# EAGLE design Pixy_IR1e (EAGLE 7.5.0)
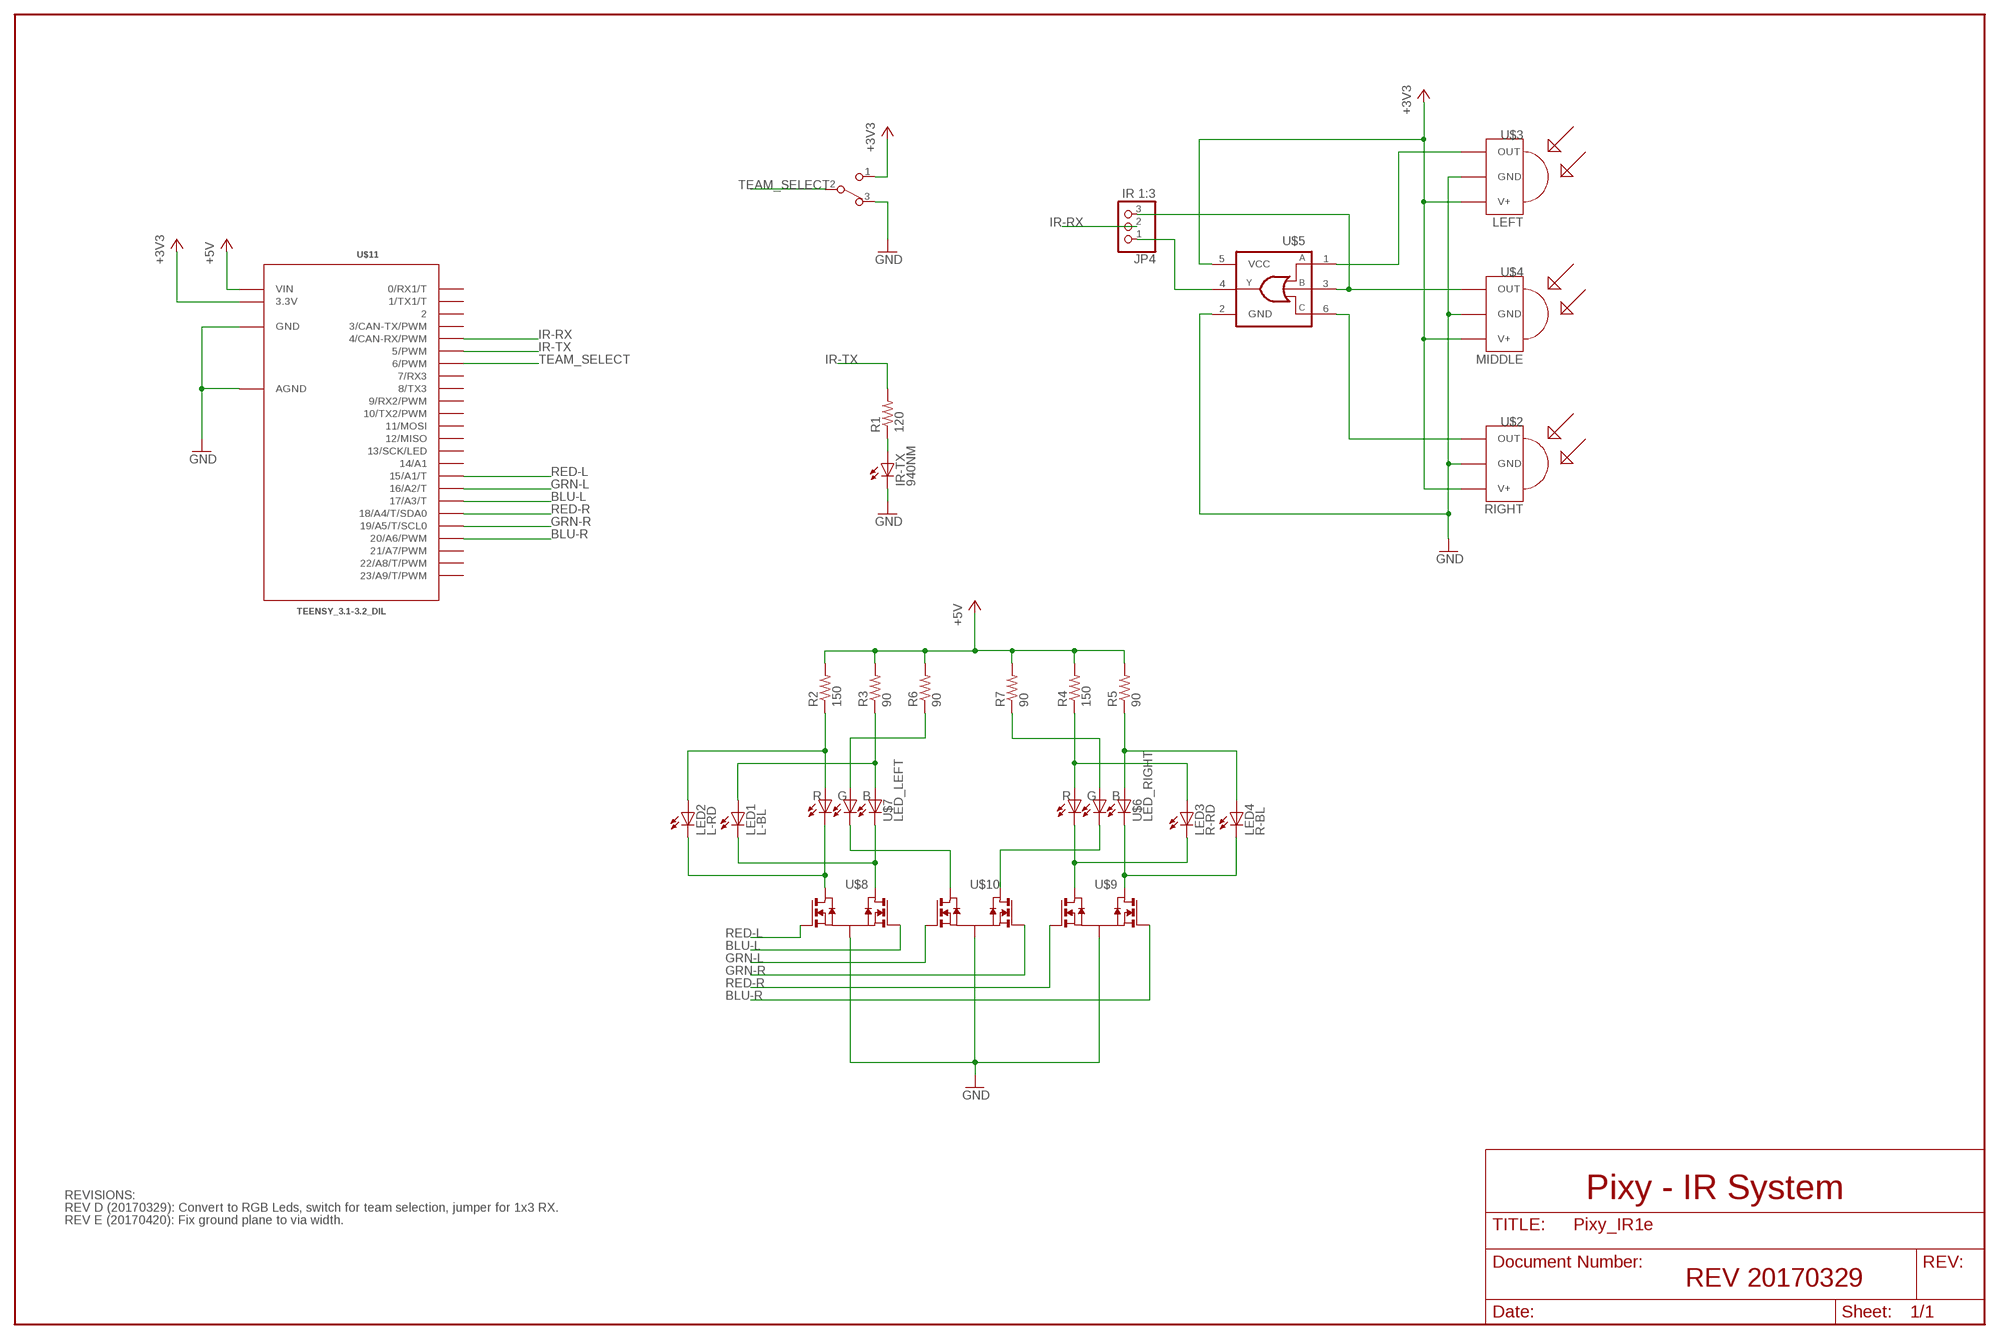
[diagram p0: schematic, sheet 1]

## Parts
IR-TX  940NM  LED5MM  [LED5MM]
JP4  IR 1:3  PINHD-1X3  [1X03]
LED1  L-BL  LED5MM  [LED5MM]
LED2  L-RD  LED5MM  [LED5MM]
LED3  R-RD  LED5MM  [LED5MM]
LED4  R-BL  LED5MM  [LED5MM]
R1  120  R-US_R1206  [R1206]
R2  150  R-US_R1206  [R1206]
R3  90  R-US_R1206  [R1206]
R4  150  R-US_R1206  [R1206]
R5  90  R-US_R1206  [R1206]
R6  90  R-US_R1206  [R1206]
R7  90  R-US_R1206  [R1206]
SW1  TEAM  CAS-120CAS-120B1  [CAS-120B1]
U$2  RIGHT  TSOP3X  [TSOP18XX]
U$3  LEFT  TSOP3X  [TSOP18XX]
U$4  MIDDLE  TSOP3X  [TSOP18XX]
U$5  SN74LVC1G332SOT23-6  [SOT23-6]
U$6  LED_RIGHT  LED_RGB_6SMD  [6-PLCC]
U$7  LED_LEFT  LED_RGB_6SMD  [6-PLCC]
U$8  QS5K2TR  [SOT-23-5]
U$9  QS5K2TR  [SOT-23-5]
U$10  QS5K2TR  [SOT-23-5]
U$11  TEENSY_3.1-3.2_DIL  [TEENSY_3.0-3.2&LC_DIL]

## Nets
+3V3: SW1.1 U$2.VCC(V+) U$3.VCC(V+) U$4.VCC(V+) U$5.5(VCC) U$11.3.3V
+5V: R2.2 R3.2 R4.2 R5.2 R6.2 R7.2 U$11.VIN
BLU-L: U$8.3(G2) U$11.17/A3(17/A3/T)
BLU-R: U$9.3(G2) U$11.20/A6(20/A6/PWM)
GND [ground]: IR-TX.K(C) SW1.3 U$2.GND U$3.GND U$4.GND U$5.2(GND) U$8.2(S) U$9.2(S) U$10.2(S) U$11.AGND U$11.GND
GRN-L: U$10.1(G1) U$11.16/A2(16/A2/T)
GRN-R: U$10.3(G2) U$11.19/A5(19/A5/T/SCL0)
IR-RX: JP4.2 U$11.4(4/CAN-RX/PWM)
IR-TX: R1.2 U$11.5(5/PWM)
N$1: U$2.OUT U$5.6(C)
N$2: U$3.OUT U$5.1(A)
N$3: LED2.A R2.1 U$7.P$1(A1)
N$4: LED1.A R3.1 U$7.P$3(A3)
N$5: R6.1 U$7.P$2(A2)
N$6: U$7.P$5(C2) U$10.5(D1)
N$8: JP4.3 U$4.OUT U$5.3(B)
N$9: JP4.1 U$5.4(Y)
N$10: IR-TX.A R1.1
N$19: LED1.K(C) U$7.P$4(C3) U$8.4(D2)
N$20: LED2.K(C) U$7.P$6(C1) U$8.5(D1)
N$25: LED3.A R4.1 U$6.P$1(A1)
N$26: LED4.A R5.1 U$6.P$3(A3)
N$28: R7.1 U$6.P$2(A2)
N$29: LED3.K(C) U$6.P$6(C1) U$9.5(D1)
N$30: LED4.K(C) U$6.P$4(C3) U$9.4(D2)
N$31: U$6.P$5(C2) U$10.4(D2)
RED-L: U$8.1(G1) U$11.15/A1(15/A1/T)
RED-R: U$9.1(G1) U$11.18/A4(18/A4/T/SDA0)
TEAM_SELECT: SW1.2 U$11.6(6/PWM)
Unconnected: U$11.0(0/RX1/T) U$11.1(1/TX1/T) U$11.2 U$11.3(3/CAN-TX/PWM) U$11.7(7/RX3) U$11.8(8/TX3) U$11.9(9/RX2/PWM) U$11.10(10/TX2/PWM) U$11.11(11/MOSI) U$11.12(12/MISO) U$11.13(13/SCK/LED) U$11.14/A0(14/A1) U$11.21/A7(21/A7/PWM) U$11.22/A8(22/A8/T/PWM) U$11.23/A9(23/A9/T/PWM)

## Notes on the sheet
- REVISIONS: | Pixy - IR System
- REV D (20170329): Convert to RGB Leds, switch for team selection, jumper for 1x3 RX.
- REV E (20170420): Fix ground plane to via width.
- REV 20170329

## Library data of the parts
IR-TX LED1-LED4 = led:LED: LED
JP4 = pinhead:PINHD-1X3: PIN HEADER
R1-R7 = resistor:R-US_: RESISTOR, American symbol
SW1 = Switch2:CAS-120: CAS-120 surface mount type slide switch Producted by COPAL ELECTRONICS Store Information : Digi-Key : http://search.digikey.com/scripts/DkSearch/dksus.dll?Detail&name=CAS120GCT-ND
U$2-U$4 = _Loper:TSOP3X: IR Receiver and Demodulator
U$5 = 74LV:SN74LVC1G332: OR GATE 3-INPUT
U$6 U$7 = _Loper:LED_RGB_6SMD
U$8-U$10 = _Loper:QS5K2TR: MOSFET 2N-CH
U$11 = Teensy_3_and_LC_Series_Boards_v1.4:TEENSY_3.1-3.2_DIL: Teensy 3.1 or 3.2 in a DIL Layout.

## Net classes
0 default: width 0.406 mm
1 ground: width 0.61 mm

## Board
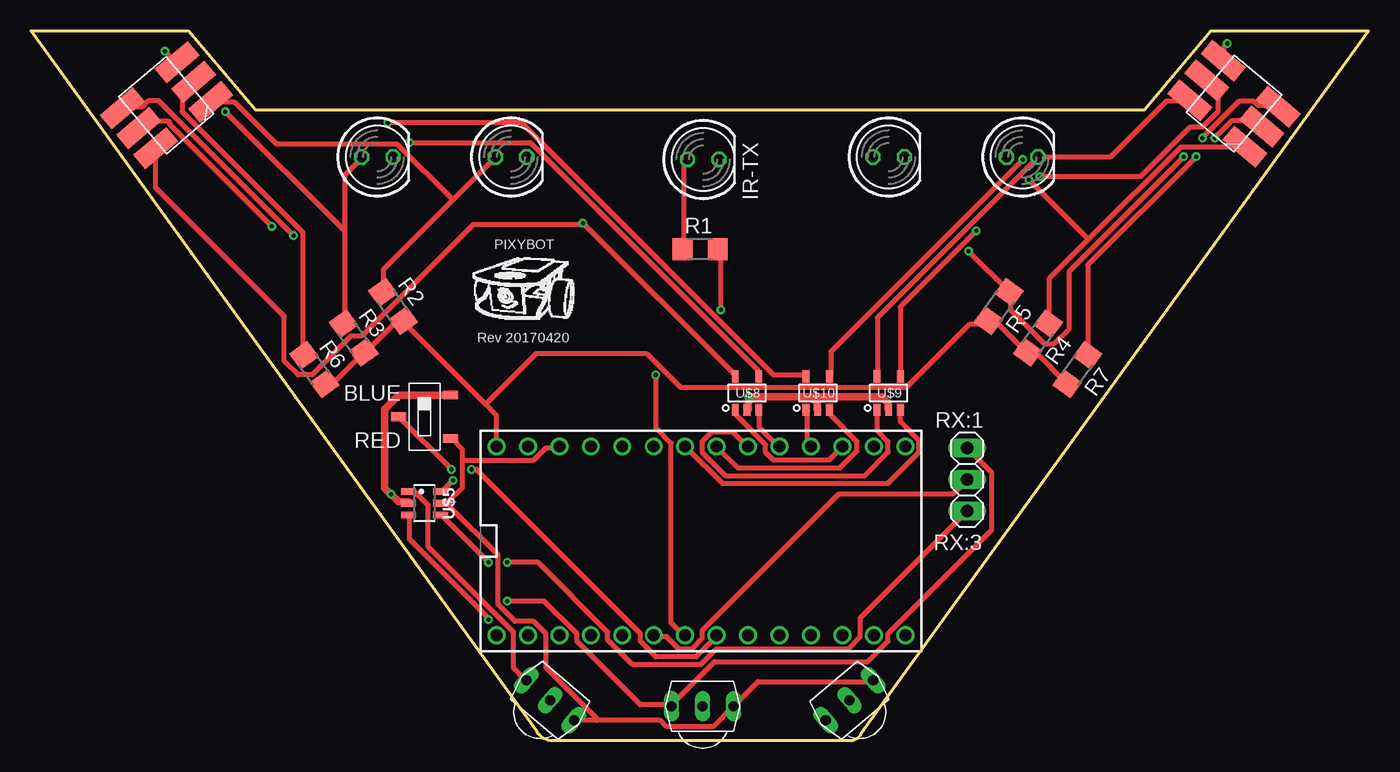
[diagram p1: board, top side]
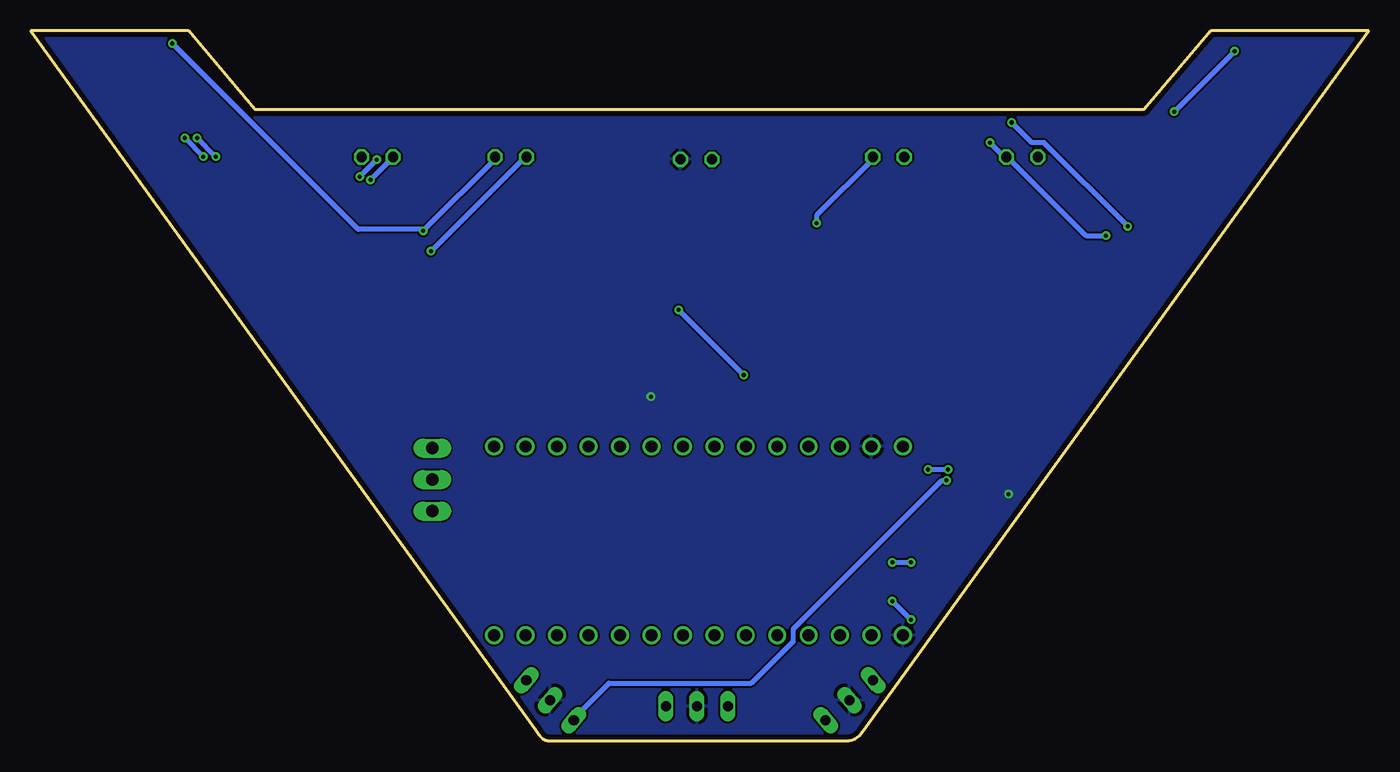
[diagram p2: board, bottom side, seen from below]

Size 107.98 x 57.28 mm. Coordinates in mm from the lower left corner, seen from the top.
Outline: 0,57.28 12.72,57.28 18.12,50.93 89.87,50.93 95.26,57.28 107.98,57.28 67.22,0.83 66.98,0.5 arc-54 66.2,0 42.06,0 arc-54 40.84,0.72 0.01,57.27
Copper layers (1*16): Top 0.0356mm / dielectric 1.5011mm / Bottom 0.0356mm
Design rules "oshpark-2layer": minimum track width 6mil, minimum drill 13mil, track to track 6mil, track to pad 6mil, pad to pad 6mil, via to via 6mil, smd to smd 6mil, copper to edge 15mil, drill to drill 6mil, minimum pad ring 7mil, minimum via ring 7mil, stop-mask expansion 2.5mil, vias tented up to drill 0mil, thermal gap 10mil

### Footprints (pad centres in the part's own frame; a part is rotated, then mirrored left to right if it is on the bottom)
LED5MM = drill 0.813 octagon: A -1.27,0; K 1.27,0
1X03 = drill 1.016 long: 1 -2.54,0; 2 0,0; 3 2.54,0
R1206 = smd 1.6 x 1.803: 1 -1.422,0; 2 1.422,0
CAS-120B1 = smd 0.7 x 1.2: 1 -1.75,-2.1; 2 0,2.1; 3 1.75,-2.1
TSOP18XX = drill 0.813 long: GND -0.001,-0.027; OUT -2.501,-0.027; VCC 2.499,-0.027
SOT23-6 = smd 0.55 x 1.2: 1 -0.95,-1.3; 2 0,-1.3; 3 0.95,-1.3; 4 0.95,1.3; 5 0,1.3; 6 -0.95,1.3
6-PLCC = smd 3.5 x 1.5: P$1 -2.77,2.41; P$2 -2.77,0.29; P$3 -2.77,-1.78; P$4 3.03,-1.78; P$5 3.03,0.29; P$6 3.03,2.41
SOT-23-5 = smd 1 x 0.55: 1 -1.35,0.95; 2 -1.35,0; 3 -1.35,-0.95; 4 1.35,-0.95; 5 1.35,0.95
TEENSY_3.0-3.2&LC_DIL = drill 0.965: 0 -7.62,13.97; 1 -7.62,11.43; 2 -7.62,8.89; 3 -7.62,6.35; 3.3V 7.62,11.43; 4 -7.62,3.81; 5 -7.62,1.27; 6 -7.62,-1.27; 7 -7.62,-3.81; 8 -7.62,-6.35; 9 -7.62,-8.89; 10 -7.62,-11.43; 11 -7.62,-13.97; 12 -7.62,-16.51; 13 7.62,-16.51; 14/A0 7.62,-13.97; 15/A1 7.62,-11.43; 16/A2 7.62,-8.89; 17/A3 7.62,-6.35; 18/A4 7.62,-3.81; 19/A5 7.62,-1.27; 20/A6 7.62,1.27; 21/A7 7.62,3.81; 22/A8 7.62,6.35; 23/A9 7.62,8.89; AGND 7.62,13.97; GND -7.62,16.51; VIN 7.62,16.51

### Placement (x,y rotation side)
IR-TX  54.27,46.91 0 top
JP4  75.58,21.07 90 top
LED1  27.96,47.11 0 top
LED2  38.75,47.11 0 top
LED3  80.03,47.11 0 top
LED4  69.23,47.11 0 top
R1  54.02,39.67 0 top
R2  29.23,35.05 306 top
R3  26.05,32.51 306 top
R4  81.3,32.51 234 top
R5  78.12,35.05 234 top
R6  22.88,29.96 306 top
R7  84.47,29.96 234 top
SW1  31.77,26.16 90 top
U$2  66.06,3.3 40 top
U$3  41.93,3.3 320 top
U$4  54.22,2.81 0 top
U$5  31.77,19.17 270 top
U$6  97.42,51.58 140 top
U$7  10.83,51.62 220 top
U$8  57.8,28.06 90 top
U$9  69.23,28.06 90 top
U$10  63.52,28.06 90 top
U$11  54.09,16.13 90 top

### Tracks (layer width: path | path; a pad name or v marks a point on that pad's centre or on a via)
+3V3
  Top 0.406: 33.69,19.27 33.19,19.27 U$5.5 | 33.69,19.27 34.81,20.39 34.81,22.64 | 34.81,22.64 34.81,23.52 33.94,24.39 SW1.1 | 34.81,22.64 40.56,22.64 41.56,23.64 42.56,23.64 U$11.3.3V | 45.69,1.65 50.81,1.65 51.31,1.15 55.06,1.15 56.69,2.77 U$4.VCC 56.81,2.9 58.69,4.77 67.94,4.77 U$2.VCC | 45.69,1.65 43.94,1.65 U$3.VCC | 33.69,19.27 33.81,19.14 33.81,18.89 37.69,15.02 37.69,11.02 39.06,9.64 40.56,9.64 41.56,8.64 41.56,5.89 45.69,1.77 45.69,1.65
+5V
  Top 0.406: R7.2 83.56,28.89 81.19,31.27 80.56,31.27 R4.2 80.31,31.39 77.94,33.77 77.31,33.77 R5.2 77.19,33.65 75.81,33.65 70.69,28.52 52.44,28.52 49.69,31.27 40.81,31.27 36.69,27.14 | R6.2 23.81,28.89 24.44,28.89 26.81,31.27 R3.2 27.06,31.39 29.44,33.77 30.06,33.77 R2.2 30.19,33.65 36.69,27.14 | 36.69,27.14 37.56,26.27 37.56,23.77 U$11.VIN
BLU-L
  Top 0.406: U$8.3 58.81,26.64 58.81,25.27 60.31,23.77 U$11.17/A3
BLU-R
  Top 0.406: U$9.3 70.19,26.64 70.19,25.77 71.69,24.27 71.69,23.27 69.19,20.77 55.81,20.77 52.94,23.64 U$11.20/A6
GND  (via drill 0.33)
  Top 0.61: U$5.2 30.44,19.27 29.69,19.27 v29.06,19.89 28.56,20.39 28.56,26.77 29.69,27.89 33.81,27.89 SW1.3 | 57.94,27.52 57.94,26.77 U$8.2 | 57.94,27.52 58.19,27.77 62.94,27.77 | 62.94,27.77 63.44,27.27 63.44,26.77 U$10.2 | 62.94,27.77 68.69,27.77 69.19,27.27 69.19,26.77 U$9.2 | v57.94,27.77 57.94,27.52
  pour Bottom: 0.1,57.21 12.69,57.2 18.12,50.92 89.87,50.92 95.27,57.27 107.97,57.27 67.04,0.6 66.11,-0.01 41.94,-0.01 40.98,0.56
GRN-L
  Top 0.406: U$10.1 62.69,26.64 62.69,24.02 62.94,23.77 U$11.16/A2
GRN-R
  Top 0.406: U$10.3 64.56,26.64 64.56,26.27 66.69,24.14 66.69,23.39 65.31,22.02 57.06,22.02 55.44,23.64 U$11.19/A5
IR-RX
  Top 0.406: U$11.4 50.31,8.39 51.31,8.39 52.31,7.39 53.31,7.39 54.19,8.27 54.19,8.89 65.19,19.89 74.44,19.89 75.56,21.02 JP4.2
IR-TX  (via drill 0.33)
  Top 0.406: v55.69,34.77 55.69,39.52 R1.2 | v50.44,29.52 50.44,25.27 51.69,24.02 51.69,9.52 52.69,8.52 U$11.5
  Bottom 0.406: v50.44,29.52 v55.69,34.77
N$1  (via drill 0.33)
  Top 0.406: v34.06,21.02 33.19,20.14 U$5.6
  Bottom 0.406: v34.06,21.02 34.44,21.02 46.44,9.02 46.44,8.02 49.81,4.64 61.31,4.64 64.19,1.77 U$2.OUT
N$2
  Top 0.406: U$5.1 30.56,20.02 31.06,20.02 32.06,19.02 32.06,15.64 38.94,8.77 38.94,5.89 39.94,4.89 U$3.OUT
N$3
  Top 0.406: 34.06,43.65 37.44,47.02 LED2.A | 34.06,43.65 28.44,38.02 28.44,36.27 R2.1 | 34.06,43.65 29.56,48.15 19.81,48.15 16.44,51.52 14.56,51.52 U$7.P$1
N$4  (via drill 0.33)
  Top 0.406: 25.31,41.27 25.31,45.65 26.69,47.02 LED1.A | 25.31,41.27 25.31,33.77 R3.1 | v10.81,55.65 11.69,54.77 U$7.P$3 | v15.69,50.77 25.19,41.27 25.31,41.27
  Bottom 0.406: v15.69,50.77 v10.81,55.65
N$5
  Top 0.406: R6.1 21.94,31.14 21.94,41.02 12.19,50.77 12.19,52.27 13.06,53.15 U$7.P$2
N$6  (via drill 0.33)
  Top 0.406: v28.81,49.9 39.56,49.9 59.94,29.52 62.56,29.52 U$10.5 | v19.44,41.52 11.19,49.77 11.19,49.9 11.06,50.02 9.31,50.02 8.81,49.52 U$7.P$5
  Bottom 0.406: v28.81,49.9 27.19,48.27 26.19,48.27 v19.44,41.52
N$8  (via drill 0.33)
  Top 0.406: v36.94,9.77 36.94,9.89 30.56,16.27 30.56,18.14 U$5.3 | v38.44,11.27 41.44,11.27 44.06,8.64 44.06,8.02 49.19,2.9 51.69,2.9 U$4.OUT 51.81,3.02 55.19,6.39 67.56,6.39 69.19,8.02 69.19,8.64 77.56,17.02 77.56,21.64 75.69,23.52 JP4.3
  Bottom 0.406: v38.44,11.27 v36.94,9.77
N$9  (via drill 0.33)
  Top 0.406: v36.94,14.39 33.19,18.14 U$5.4 | v38.44,14.39 40.94,14.39 46.56,8.77 46.56,8.14 48.56,6.14 54.06,6.14 55.31,7.39 65.94,7.39 66.94,8.39 66.94,9.89 75.56,18.52 JP4.1
  Bottom 0.406: v38.44,14.39 v36.94,14.39
N$10
  Top 0.406: R1.1 52.69,39.77 52.69,46.52 52.94,46.77 IR-TX.A
N$19  (via drill 0.33)
  Top 0.406: v30.56,48.27 40.31,48.27 58.69,29.89 58.69,29.52 U$8.4 | v21.19,40.77 10.31,51.65 9.44,51.65 8.94,51.15 7.44,51.15 U$7.P$4
  Bottom 0.406: v30.56,48.27 29.31,47.02 LED1.K 29.06,47.02 22.81,40.77 v21.19,40.77
N$20  (via drill 0.33)
  Top 0.406: U$8.5 56.81,29.52 v44.56,41.77 44.44,41.65 35.69,41.65 26.69,32.65 25.81,32.65 22.69,29.52 21.56,29.52 20.44,30.64 20.44,34.27 10.06,44.65 10.06,47.77 U$7.P$6
  Bottom 0.406: v44.56,41.77 44.56,42.4 39.94,47.02 LED2.K
N$25  (via drill 0.33)
  Top 0.406: 85.38,40.46 92.81,47.9 97.94,47.9 U$6.P$1 | 85.38,40.46 82.19,37.27 82.19,33.77 R4.1 | 85.38,40.46 v80.56,45.27
  Bottom 0.406: v80.56,45.27 78.81,47.02 LED3.A
N$26  (via drill 0.33)
  Top 0.406: v75.69,39.52 78.94,36.27 R5.1 79.06,36.02 79.06,34.77 81.81,32.02 82.56,32.02 83.81,33.27 83.81,37.9 v93.06,47.15 | v94.56,48.65 97.56,51.65 98.69,51.65 99.06,51.27 100.56,51.27 U$6.P$3
  Bottom 0.406: v75.69,39.52 68.06,47.15 LED4.A | v93.06,47.15 v94.56,48.65
N$28  (via drill 0.33)
  Top 0.406: v94.06,47.15 85.31,38.4 85.31,31.14 R7.1 | v95.56,48.65 96.94,50.02 98.94,50.02 99.31,49.65 U$6.P$2
  Bottom 0.406: v95.56,48.65 v94.06,47.15
N$29
  Top 0.406: U$9.5 68.31,29.52 68.31,34.15 81.19,47.02 LED3.K 81.44,47.15 87.19,47.15 91.69,51.65 93.44,51.65 U$6.P$6
N$30  (via drill 0.33)
  Top 0.406: v76.31,41.15 70.19,35.02 70.19,29.52 U$9.4 | v96.56,56.27 96.31,56.02 96.31,54.9 U$6.P$4
  Bottom 0.406: LED4.K 70.44,47.02 v76.31,41.15 76.44,41.27 81.56,41.27 v96.56,56.27
N$31  (via drill 0.33)
  Top 0.406: v80.06,46.9 64.56,31.39 64.56,29.52 U$10.4 | v81.44,45.52 89.56,45.52 93.56,49.52 94.56,49.52 95.81,50.77 95.81,52.4 94.94,53.27 U$6.P$5
  Bottom 0.406: v81.44,45.52 v80.06,46.9
RED-L
  Top 0.406: U$8.1 56.94,26.64 56.94,26.27 59.31,23.89 59.31,23.27 59.94,22.64 64.44,22.64 65.44,23.64 U$11.15/A1
RED-R
  Top 0.406: U$9.1 68.31,26.64 68.31,25.02 69.19,24.14 69.19,23.27 67.31,21.39 56.06,21.39 54.19,23.27 54.19,24.14 54.94,24.89 56.69,24.89 57.81,23.77 U$11.18/A4
TEAM_SELECT  (via drill 0.33)
  Top 0.406: v33.94,21.89 29.69,26.14 SW1.2 | v35.56,21.89 35.94,21.89 49.19,8.64 49.19,8.02 50.44,6.77 53.69,6.77 55.31,8.39 U$11.6
  Bottom 0.406: v35.56,21.89 v33.94,21.89

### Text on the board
tPlace: PIXYBOT | Rev 20170420 | BLUE | RED | RX:1 | RX:3

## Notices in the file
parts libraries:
74LV: Copyright (C) 2008, Bob Starr
